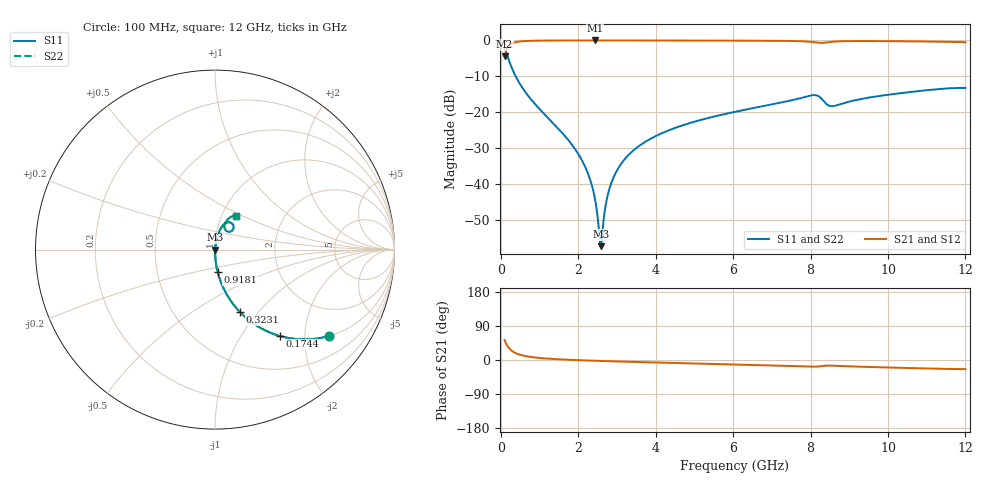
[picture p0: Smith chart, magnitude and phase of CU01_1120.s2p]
! S-parameter model data by Modelithics Inc. support@modelithics.com 813-866-6335 Tampa FL USA
! S-Parameter data specifications:
! Substrate: 20-mil Rogers, substrate thickness, H=0.508mm, Dielectric constant, Er=3.75
! PCB Mounting Pad Footprint: Pad width, PadW=0.35mm , Pad length, PadL=0.30mm , Pad gap, PadG (edge-to-edge)=0.25mm , Reference planes=0.85mm apart
! Created Tue May  8 14:01:25 2018
# hz S ma R 50
! 2 Port Network Data from SP1.SP block
! freq  magS11  angS11  magS21  angS21  magS12  angS12  magS22  angS22
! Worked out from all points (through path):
!   801 points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, 100 MHz to 12 GHz, reference 50 ohm
!   highest |S21| = -0.01 dB at 2.435 GHz (marker M1); lowest = -4.4 dB at 100 MHz (marker M2)
!   group delay of S21, straight-line fit = 8.15 ps
!   lowest |S11| = -57.2 dB at 2.584 GHz (marker M3), VSWR 1.00, Z = 50.1 - j0.00055 ohm
!   |S11| at or under -10 dB: 387.2 MHz to end of sweep
!   |S22| runs from -57.2 to -2.0 dB; largest |S21 - S12| = 0
!   S11 on the Smith chart (normalised r, x): 100 MHz: 1.00, -2.63; 174.4 MHz: 1.00, -1.50; 323.1 MHz: 1.00, -0.80; 918.1 MHz: 1.00, -0.25; 12 GHz: 1.17, +0.45
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1e8  0.7966 -37.3  0.6041 52.7  0.6041 52.7  0.7966 -37.3
1.74375e8  0.6018 -53.1  0.7982 36.8  0.7982 36.8  0.6018 -53.1
3.23125e8  0.3731 -68.3  0.9272 21.6  0.9272 21.6  0.3731 -68.3
5.31375e8  0.2315 -77.0  0.9721 12.9  0.9721 12.9  0.2315 -77.0
9.18125e8  0.1247 -83.3  0.9913 6.3  0.9913 6.3  0.1247 -83.3
1.7065e9  0.04364 -87.7  0.9979 0.8  0.9979 0.8  0.04364 -87.7
2.09325e9  0.02173 -87.5  0.9985 -0.8  0.9985 -0.8  0.02173 -87.5
2.3015e9  0.01193 -85.3  0.9986 -1.6  0.9986 -1.6  0.01193 -85.3
2.435375e9  0.006182 -79.5  0.9986 -2.0  0.9986 -2.0  0.006182 -79.5
2.5395e9  0.002209 -54.1  0.9986 -2.4  0.9986 -2.4  0.002209 -54.1
2.584125e9  0.00138 -0.2  0.9986 -2.5  0.9986 -2.5  0.00138 -0.2
2.62875e9  0.002286 49.9  0.9986 -2.7  0.9986 -2.7  0.002286 49.9
2.703125e9  0.004891 70.4  0.9985 -2.9  0.9985 -2.9  0.004891 70.4
2.7775e9  0.007615 76.1  0.9985 -3.1  0.9985 -3.1  0.007615 76.1
3.0155e9  0.01608 80.9  0.9983 -3.9  0.9983 -3.9  0.01608 80.9
3.432e9  0.02976 81.9  0.9979 -5.0  0.9979 -5.0  0.02976 81.9
4.071625e9  0.04881 81.2  0.997 -6.8  0.997 -6.8  0.04881 81.2
6.05e9  0.1017 76.9  0.9922 -11.7  0.9922 -11.7  0.1017 76.9
8.04325e9  0.1729 61.1  0.9515 -17.6  0.9515 -17.6  0.1729 61.1
8.563875e9  0.1219 58.7  0.9588 -15.0  0.9588 -15.0  0.1219 58.7
1.002162e10  0.1762 67.7  0.9766 -19.9  0.9766 -19.9  0.1762 67.7
1.2e10  0.2187 57.6  0.9446 -24.1  0.9446 -24.1  0.2187 57.6
